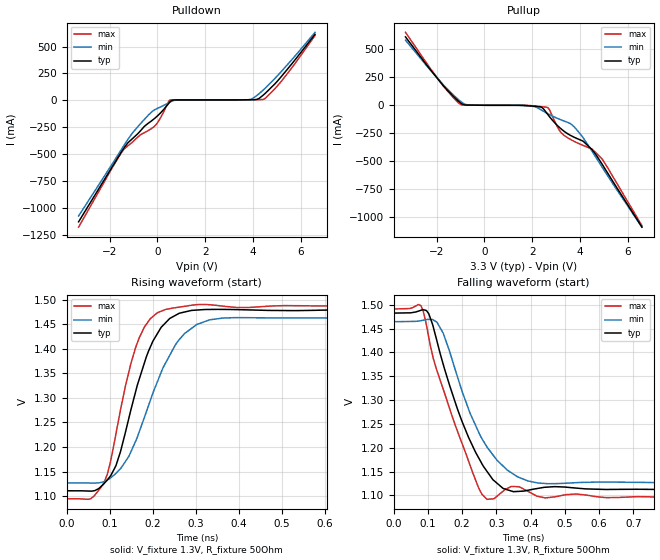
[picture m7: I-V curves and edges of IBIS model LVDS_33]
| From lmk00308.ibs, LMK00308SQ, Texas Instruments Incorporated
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|   Model LVDS_33
[Model]   LVDS_33
Model_type   Output
Polarity   Non-Inverting
Rref =   50.0000
Vref =   1.3
Vmeas =   1.3
|   typ   min   max
|   Nom   Weak   Strong
C_comp   0.6362pF   0.6362pF   0.8920pF
|Output in low   Nom   Weak   Strong
|C_Comp   0.6362pF   0.6362pF   0.8920pF
|Output in High   Nom   Strong   Weak
|C_Comp   1.1227pF   1.0238pF   1.1227pF
[Voltage Range]   3.3   3.125   3.465
[Temperature Range]   45   125   -40
[Pullup Reference]   3.3   3.125   3.465
[Pulldown Reference]   0   -0   0
[Power Clamp Reference]   3.3   3.125   3.465
[GND Clamp Reference]   0   0   0
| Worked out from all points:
|   slope of the pulldown table from 0 to 0.495 V, typ, clamps not added: 4.02 ohm
|   slope of the pullup table from 0 to 0.495 V, typ, clamps not added: 3.09 kohm
|   falling waveform, V_fixture 1.3V, R_fixture 50Ohm: 20-80 % time 111ps typ, 114ps min, 110ps max; typ from 1.48 V to 1.11 V
|   rising waveform, V_fixture 1.3V, R_fixture 50Ohm: 20-80 % time 72.9ps typ, 94.3ps min, 60.5ps max; typ from 1.11 V to 1.48 V
[Pulldown]
|   Voltage   I(typ)   I(min)   I(max)
-3.3V     -1.13A     -1.076A    -1.18A
-1.523V   -485mA     -462mA     -491.1mA
-1.053V   -357.7mA   -305.3mA   -390.3mA
-389.4mV  -213.8mA   -139.5mA   -281.5mA
-67.65mV  -158.3mA   -81.95mA   -228.5mA
491.7mV   -22.58mA   -20.78mA   -2.718mA
699.6mV   3.699mA    -82.36uA   4.119mA
3.887V    5.712mA    8.578mA    5.709mA
4.145V    7.656mA    42.72mA    6.203mA
4.471V    57.42mA    105.1mA    12.56mA
5.214V    229.4mA    275.9mA    185.2mA
6.595V    614.5mA    632.9mA    603.4mA
[Pullup]
|   Voltage   I(typ)   I(min)   I(max)
-3.3V     611.5mA    582.8mA    652.4mA
-1.721V   175.9mA    184.3mA    174.1mA
-1.063V   33.17mA    47.33mA    18.02mA
-686.4mV  1.984mA    2.613mA    2.039mA
1.744V    -2.411mA   -4.408mA   -116.1uA
2.363V    -14.66mA   -39.13mA   -11.78mA
2.64V     -77.67mA   -72.85mA   -18.7mA
3.194V    -207.6mA   -128.9mA   -240mA
3.62V     -270.7mA   -166.3mA   -306.9mA
4.14V     -321.5mA   -291.2mA   -359mA
4.932V    -527.6mA   -553.9mA   -480.4mA
6.595V    -1.089A    -1.089A    -1.076A
[Ramp]
R_load = 50
|   typ   min   max
dV/dt_r   0.221632/7.28869e-11   0.202369/9.43072e-11   0.236331/6.05332e-11
dV/dt_f   0.222237/1.1072e-10   0.202369/1.14375e-10   0.237272/1.09637e-10
[Falling Waveform]
V_fixture = 1.3V
V_fixture_min = 1.3V
V_fixture_max = 1.3V
R_fixture = 50Ohm
C_fixture = 0F
|   Time   V(typ)   V(min)   V(max)
0s        1.482V     1.464V     1.491V
79.8ps    1.488V     1.467V     1.498V
102.3ps   1.481V     1.469V     1.432V
144.5ps   1.375V     1.441V     1.323V
200.3ps   1.254V     1.317V     1.208V
250ps     1.176V     1.23V      1.113V
272.5ps   1.151V     1.202V     1.092V
319.6ps   1.115V     1.162V     1.109V
422.1ps   1.115V     1.126V     1.098V
1.4ns     1.112V     1.127V     1.096V
[Rising Waveform]
V_fixture = 1.3V
V_fixture_min = 1.3V
V_fixture_max = 1.3V
R_fixture = 50Ohm
C_fixture = 0F
|   Time   V(typ)   V(min)   V(max)
0s        1.111V     1.127V     1.095V
61.98ps   1.111V     1.127V     1.099V
102.3ps   1.142V     1.138V     1.173V
124.9ps   1.191V     1.156V     1.276V
162.5ps   1.321V     1.217V     1.409V
200ps     1.415V     1.31V      1.466V
230.6ps   1.454V     1.373V     1.48V
273.8ps   1.475V     1.431V     1.486V
362.1ps   1.48V      1.463V     1.487V
1.4ns     1.48V      1.464V     1.489V
